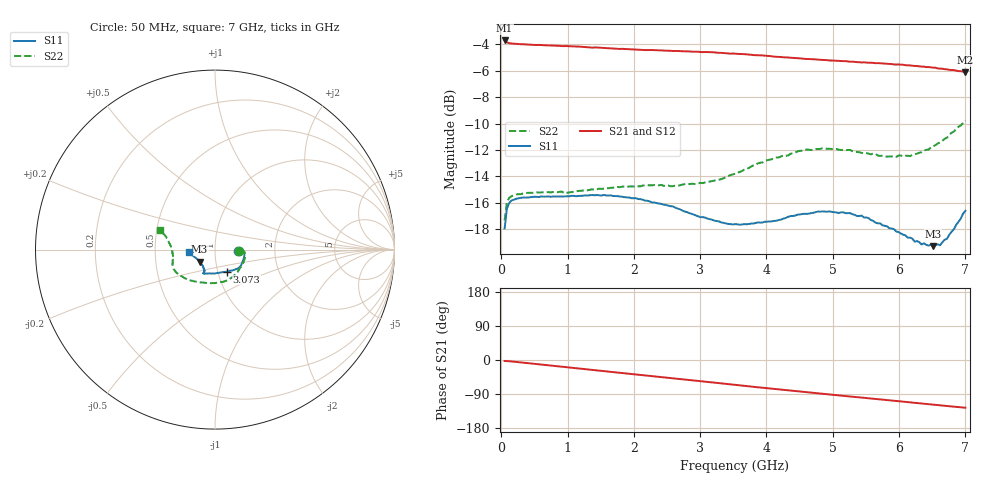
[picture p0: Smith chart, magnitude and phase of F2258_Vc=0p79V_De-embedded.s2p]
! Integrated Device Technology
! Corporate Headquarters
! 6024 Silver Creek Valley Road
! San Jose, CA 95138  USA
! Phone:  1-408-284-8200
! Toll Free:  1-800-223-1366
! Webpage:  http://www.idt.com/
! Timing and RF Division
! 515 Groton Road, Suite 102
! Westford, MA 01886-6024
! Device:  F2258
! Description: Voltage Variable RF Attenuator
! Frequency:  50.0 -  6000.00 MHz
! Package:  3x3 mm Thin QFN Plastic Package: 16 pin
! Ports:  2 RF, 2 DC
!  Pin  1  = NC
!  Pin  2  = NC
!  Pin  3  = RF2  = Port 2
!  Pin  4  = GND
!  Pin  5  = Vdd
!  Pin  6  = NC
!  Pin  7  = VCTRL
!  Pin  8  = NC
!  Pin  9  = GND
!  Pin 10  = RF1  = Port 1
!  Pin 11  = NC
!  Pin 12  = NC
!  Pin 13  = NC
!  Pin 14  = NC
!  Pin 15  = NC
!  Pin 16  = NC
! Vcntrl:  0.790 Volts
! Vdd:  +3.300 Volts
! Current:  1.133 mA
! Data:  The device was measured on a the F2258 evaluation board which has
!  individual transmission lines to the RF pins.  Data was collected
!  using a calibrated network analyzer.  The evaluation board was
!  de-embedded using a TRL calibration technique.
!  The reference plane is the edge of the package pin.
! Misc:  SN 10
!  Action Tracker AT0285
! Date Measured:  2014-12-10
! Date:  2016-01-13  MJV
! Note:
!  Integrated Device Technology supplies this data as a sample of measured
!  data at the package pin for this product.  Your particular data for this
!  product may vary.
!  Data was taken at 25 degrees C.
!  Integrated Device Technology reserves the right to change this data at anytime.
!Freq_(GHz)  S11M_(dB)  S11P_(deg)  S21M_(dB)  S21P_(deg)  S12M_(dB)  S12P_(deg)  S22M_(dB)  S22P_(deg)
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# GHz S dB R 50
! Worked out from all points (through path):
!   201 points, 50 MHz to 7 GHz, reference 50 ohm
!   highest |S21| = -3.72 dB at 50 MHz (marker M1); lowest = -6.1 dB at 7 GHz (marker M2)
!   group delay of S21, straight-line fit = 49.8 ps
!   lowest |S11| = -19.3 dB at 6.513 GHz (marker M3), VSWR 1.24, Z = 41.8 - j5.64 ohm
!   |S11| at or under -10 dB: start of sweep to end of sweep
!   |S22| runs from -17.3 to -9.8 dB; largest |S21 - S12| = 0.0016
!   S11 on the Smith chart (normalised r, x): 50 MHz: 1.29, -0.02; 3.073 GHz: 1.11, -0.28; 7 GHz: 0.74, -0.02
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0.05  -17.95 -3.7  -3.72 -2.6  -3.71 -2.6  -17.33 -4.3
0.08475  -16.44 -3.2  -3.86 -2.8  -3.86 -2.8  -15.97 -4.1
0.15425  -15.83 -3.9  -3.95 -3.8  -3.94 -3.8  -15.50 -6.4
0.5365  -15.55 -12.8  -4.06 -10.9  -4.06 -10.9  -15.20 -19.6
0.9535  -15.51 -23.2  -4.15 -18.7  -4.14 -18.7  -15.28 -34.9
1.2315  -15.46 -28.3  -4.21 -23.8  -4.21 -23.8  -15.07 -44.1
1.6485  -15.43 -34.8  -4.32 -31.3  -4.32 -31.3  -14.86 -56.2
2.37825  -16.05 -44.5  -4.47 -44.4  -4.46 -44.4  -14.68 -76.2
3.07325  -17.11 -61.2  -4.59 -57.1  -4.59 -57.1  -14.45 -100.1
3.525  -17.61 -78.4  -4.72 -65.6  -4.72 -65.6  -13.80 -118.0
4.11575  -17.36 -101.6  -4.94 -76.4  -4.94 -76.4  -12.62 -138.3
4.498  -16.88 -111.6  -5.07 -83.3  -5.08 -83.3  -12.07 -148.1
4.7065  -16.75 -113.8  -5.14 -86.9  -5.14 -86.9  -11.98 -152.2
5.2625  -16.78 -116.6  -5.33 -96.3  -5.31 -96.3  -12.00 -161.4
5.5405  -17.16 -116.2  -5.41 -101.0  -5.39 -101.0  -12.28 -166.2
5.85325  -17.92 -118.0  -5.50 -106.3  -5.49 -106.3  -12.49 -172.7
6.166  -18.63 -123.6  -5.61 -111.7  -5.61 -111.7  -12.47 -179.7
6.33975  -19.15 -130.7  -5.69 -114.8  -5.69 -114.8  -12.16 175.5
6.5135  -19.28 -142.1  -5.77 -117.8  -5.78 -117.8  -11.72 171.1
6.61775  -19.21 -148.9  -5.85 -119.5  -5.83 -119.5  -11.44 168.2
6.722  -18.72 -156.6  -5.90 -121.4  -5.91 -121.4  -11.08 165.5
7  -16.60 -174.4  -6.12 -125.9  -6.13 -125.9  -9.77 159.8
